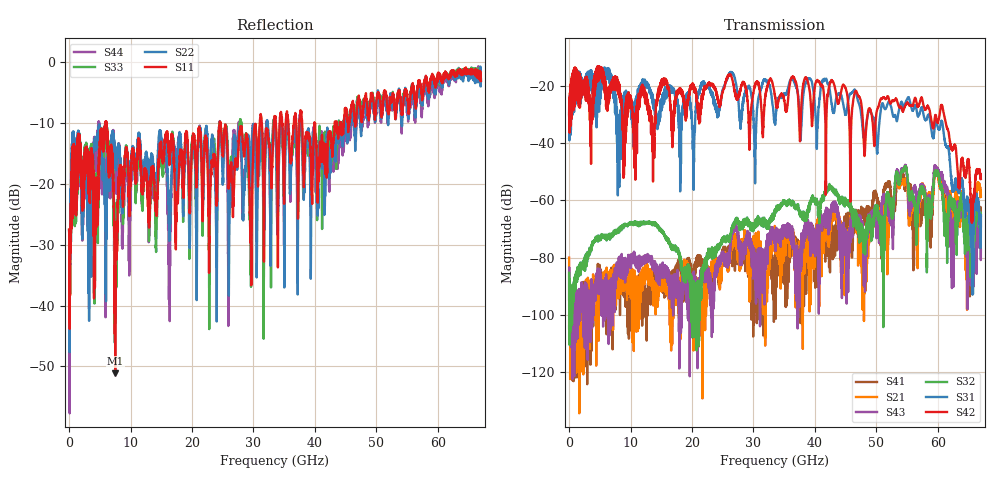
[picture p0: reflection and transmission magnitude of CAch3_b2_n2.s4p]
!Agilent Technologies,N5247A,US51170199,A.09.90.13
!Agilent N5247A: A.09.90.13
!Date: Thursday, October 18, 2018 09:27:05
!Correction: S11(Full 4 Port(1,2,3,4))
!S12(Full 4 Port(1,2,3,4))
!S13(Full 4 Port(1,2,3,4))
!S14(Full 4 Port(1,2,3,4))
!S21(Full 4 Port(1,2,3,4))
!S22(Full 4 Port(1,2,3,4))
!S23(Full 4 Port(1,2,3,4))
!S24(Full 4 Port(1,2,3,4))
!S31(Full 4 Port(1,2,3,4))
!S32(Full 4 Port(1,2,3,4))
!S33(Full 4 Port(1,2,3,4))
!S34(Full 4 Port(1,2,3,4))
!S41(Full 4 Port(1,2,3,4))
!S42(Full 4 Port(1,2,3,4))
!S43(Full 4 Port(1,2,3,4))
!S44(Full 4 Port(1,2,3,4))
!S4P File: Measurements: <S11,S12,S13,S14>,
!<S21,S22,S23,S24>,
!<S31,S32,S33,S34>,
!<S41,S42,S43,S44>:
# Hz S  dB  R 50
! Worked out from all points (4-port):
!   6701 points, 10 MHz to 67 GHz, reference 50 ohm
!   strongest paths, dB at 10 MHz, 16.76 GHz, 33.51 GHz, 50.25 GHz, 67 GHz:
!     S42: -29.9, -37.8, -23.5, -27.6, -52.5
!     S31: -30.3, -21.4, -32.7, -39.7, -65.1
!     S32: -85.3, -76.1, -64.4, -66.6, -65.3
!     S43: -94.5, -92.2, -73.3, -67.9, -77.2
!     S21: -79.9, -90.7, -72.8, -67.4, -58.5
!     S41: -104.7, -86.8, -87.6, -62.5, -69.0
!   lowest |S11| = -51.1 dB at 7.509 GHz (marker M1), VSWR 1.01, Z = 50.2 + j0.197 ohm
!   |S11| at or under -10 dB: start of sweep to 5.921 GHz; 6.065 GHz to 24.48 GHz (18.42 GHz wide, 121 % of centre); 24.67 GHz to 31.03 GHz (6.357 GHz wide, 22.8 % of centre)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
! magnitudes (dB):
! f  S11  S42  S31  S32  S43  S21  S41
! 10 MHz  -27.5  -29.9  -30.3  -85.3  -94.5  -79.9  -104.7
! 5.989 GHz  -9.7  -19.8  -14.0  -72.5  -87.7  -88.0  -84.8
! 7.509 GHz  -51.1  -19.9  -23.0  -71.4  -86.4  -87.2  -91.4
! 42.35 GHz  -11.7  -20.0  -20.8  -54.7  -65.6  -70.3  -80.2
! 51.01 GHz  -7.3  -24.3  -26.1  -71.0  -59.6  -61.8  -60.7
! 55.16 GHz  -7.0  -26.1  -24.0  -53.9  -57.5  -61.3  -53.7
! 67 GHz  -3.1  -52.5  -65.1  -65.3  -77.2  -58.5  -69.0
